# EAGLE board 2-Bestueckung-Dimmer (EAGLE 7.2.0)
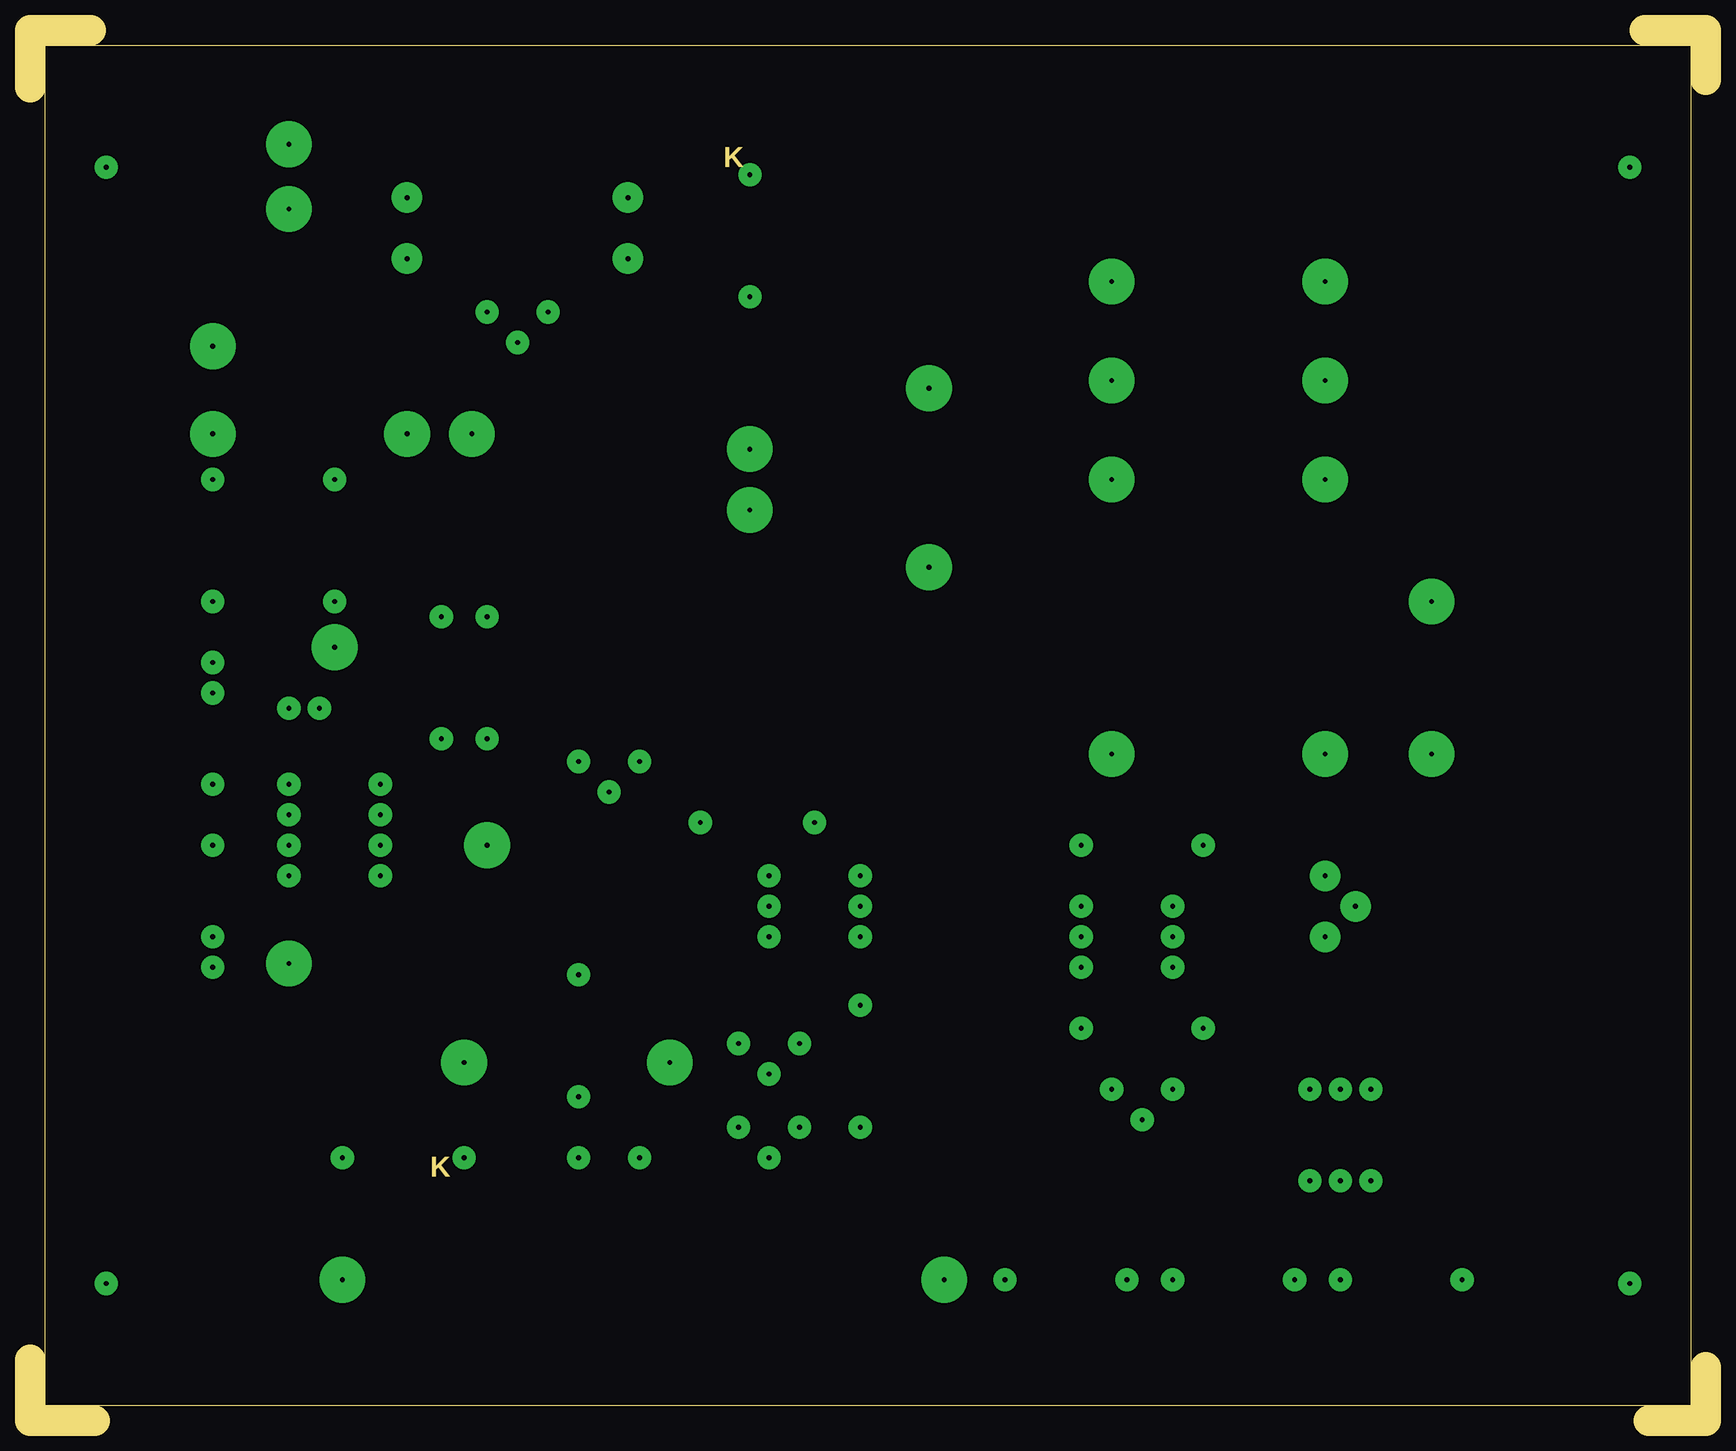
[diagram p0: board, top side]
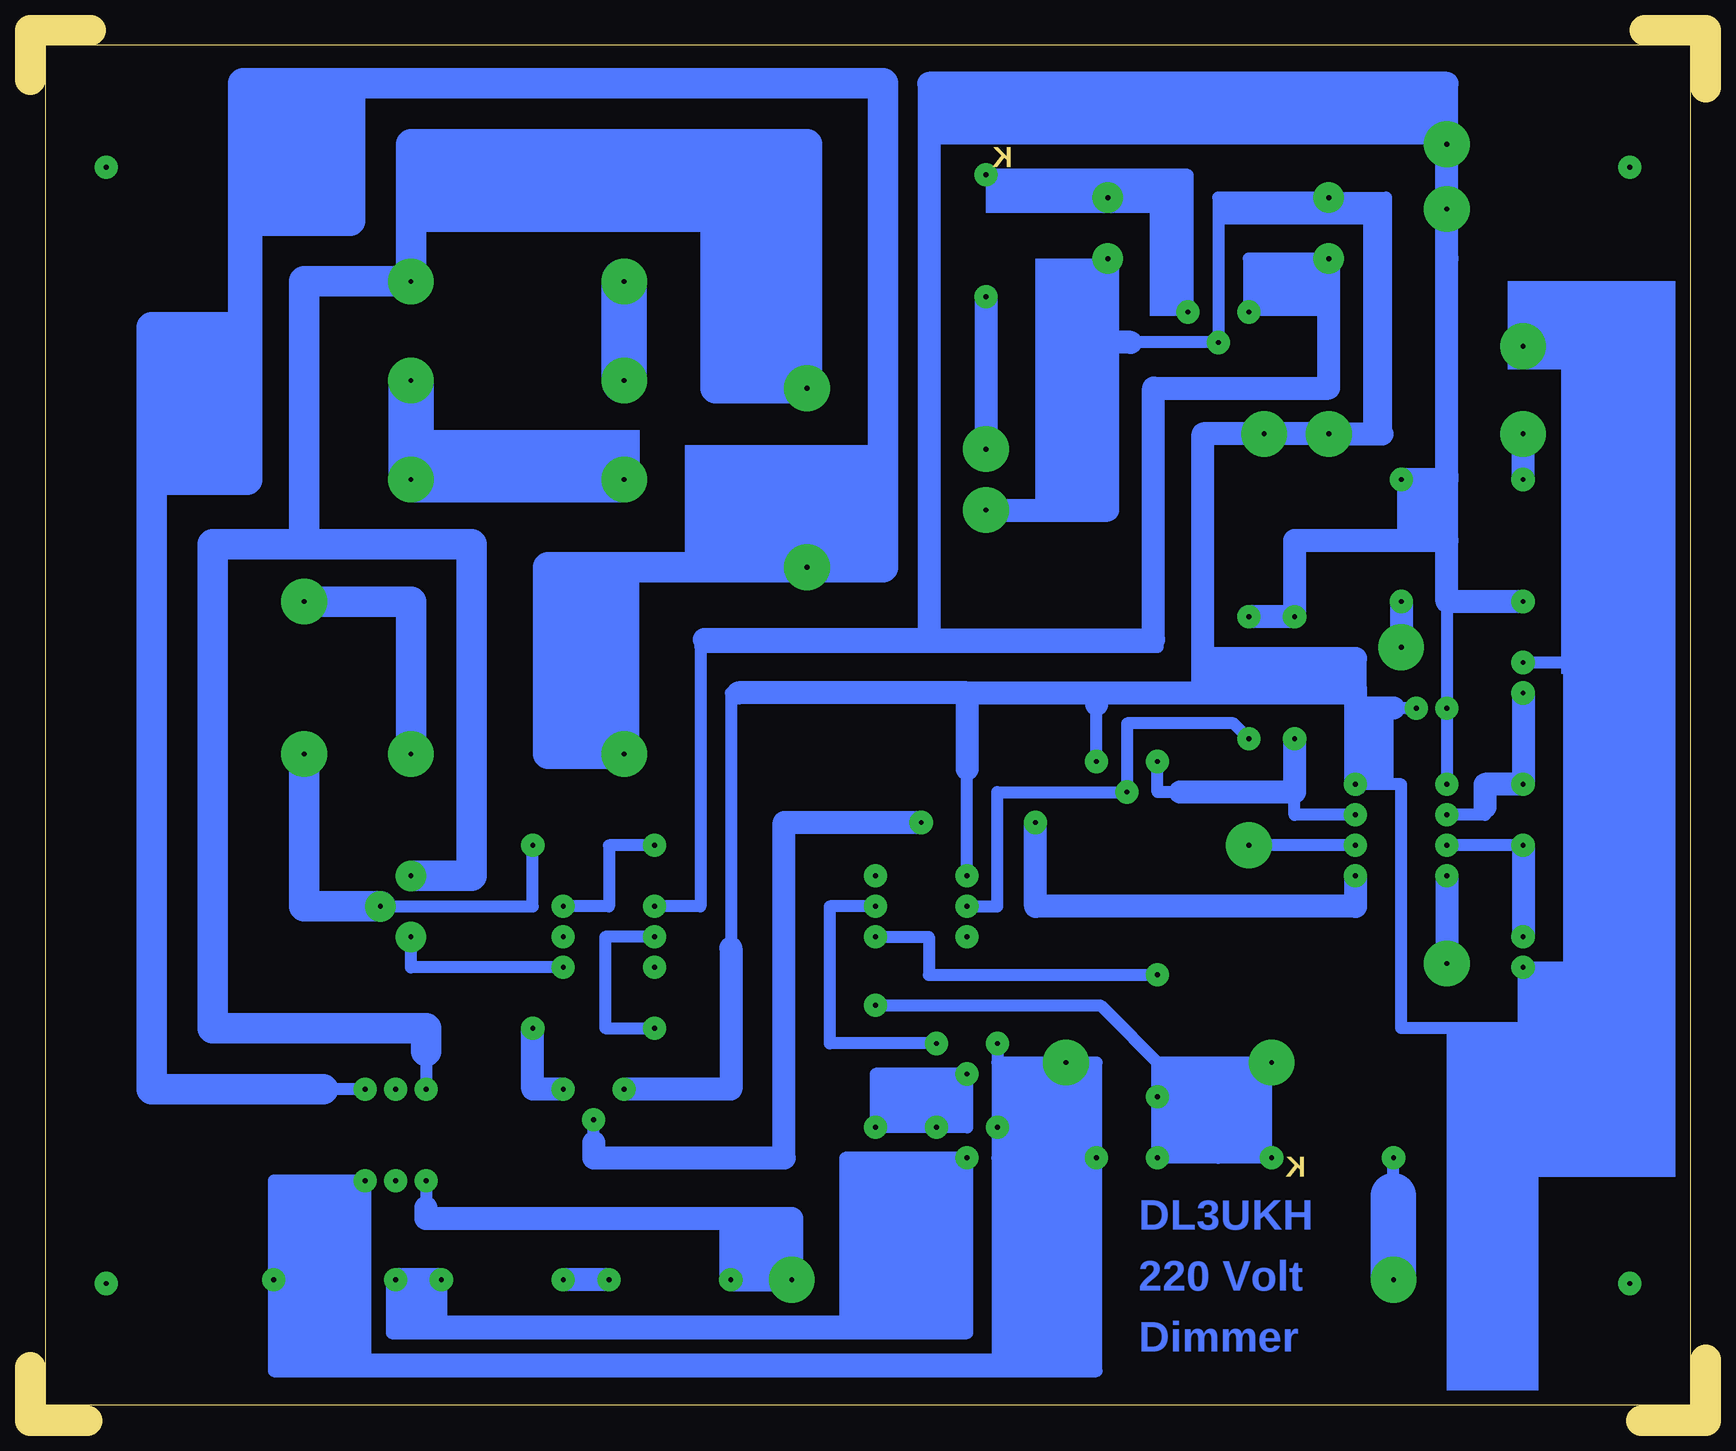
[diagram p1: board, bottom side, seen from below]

Size 139.7 x 115.89 mm. Coordinates in mm from the lower left corner, seen from the top.
Outline: 5.4,0 0.32,0
Outline: 0,0 0,5.08
Outline: 134.94,0 139.7,0 139.7,4.45
Outline: 5.08,115.89 0,115.89 0,111.12
Outline: 139.7,111.76 139.7,115.89
Outline: 134.62,115.89 139.38,115.89
Outline: 1.27,1.27 138.43,1.27 138.43,114.62 1.27,114.62 1.27,1.27
Copper layers (1*16): Top 0.035mm / dielectric 1.5mm / Bottom 0.035mm
Design rules "default": minimum track width 10mil, minimum drill 24mil, track to track 8mil, track to pad 8mil, pad to pad 8mil, via to via 8mil, smd to smd 8mil, copper to edge 40mil, drill to drill 8mil, minimum pad ring 10mil, minimum via ring 8mil, stop-mask expansion 4mil, vias tented up to drill 0mil, thermal gap 10mil

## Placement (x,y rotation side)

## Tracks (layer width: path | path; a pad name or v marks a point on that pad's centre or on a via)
S$1  (via drill 0.4 pad 1.93)
  other vias: 6.35,104.46
S$2  (via drill 0.4 pad 1.93)
  other vias: 133.35,104.46
S$3  (via drill 0.4 pad 1.93)
  other vias: 133.35,11.43
S$4  (via drill 0.4 pad 1.93)
  other vias: 6.35,11.43
S$5  (via drill 0.4 pad 2.54, 0.4 pad 3.81)
  Bottom 1.016: v110.49,42.86 97.79,42.86 97.79,47.94
  Bottom 2.54: v116.84,55.56 116.84,42.86 v110.49,42.86
S$6  (via drill 0.4 pad 1.93, 0.4 pad 2.54, 0.4 pad 3.81)
  Bottom 1.016: v38.1,92.39 38.1,96.84 v31.43,96.84 | 31.43,86.04 45.72,86.04 45.72,64.45 65.09,64.45 | 65.09,64.45 83.82,64.45 83.82,42.86 v87.63,42.86 | 65.09,64.45 65.09,65.09 65.09,111.44 64.77,111.44 | 21.59,111.44 v21.59,106.36 v21.59,100.96 21.59,96.84 | 21.59,78.74 21.59,78.42 | v21.59,53.02 v21.59,59.37 21.59,68.26 21.27,68.26
  Bottom 1.93: v15.24,68.26 21.27,68.26 | 21.59,68.26 21.59,73.34 | 21.59,73.34 34.29,73.34 34.29,66.99 v38.1,66.99 | 21.59,73.34 21.59,78.42 v25.4,78.42 | 21.59,78.74 21.59,96.84 21.59,111.44 64.77,111.44 64.77,65.09 | 64.77,65.09 65.09,65.09 83.5,65.09 | 64.77,65.09 46.04,65.09 46.04,86.04 31.43,86.04 v31.43,96.84
S$7  (via drill 0.4 pad 3.81)
  Bottom 1.016: 107.95,55.25 v107.95,55.56 | 109.54,68.26 v116.84,68.26
  Bottom 2.54: v107.95,55.56 107.95,68.26 108.9,68.26 109.54,68.26
S$8  (via drill 0.4 pad 3.81)
  Bottom 3.81: v90.17,86.68 v90.17,94.93
S$9  (via drill 0.4 pad 1.93, 0.4 pad 2.54, 0.4 pad 3.81)
  Bottom 1.016: 26.04,18.73 v26.04,21.91 | v15.24,78.42 v15.24,82.23 | 47.94,89.85 v40.64,89.85 40.64,101.92 v31.43,101.92 26.67,101.92 26.67,82.23 26.99,82.23 | v31.43,82.23 v36.83,82.23 41.91,82.23 | 80.64,60.64 81.28,60.64 81.28,39.37 | 29.21,59.37 v29.21,53.02 25.4,53.02 25.4,32.7 15.24,32.7 v15.24,37.78 11.43,37.78 11.43,63.18 v15.24,63.18 | 29.21,59.37 29.21,60.64 | v50.8,54.93 50.8,59.69 | v24.13,59.37 26.04,59.37 | 28.89,59.37 29.21,59.37 | v61.6,45.4 61.6,54.29 61.6,60.33 61.91,60.33
  Bottom 1.93: v21.59,45.4 v21.59,38.1 | v15.24,78.42 15.24,82.55 | 61.6,60.64 61.6,54.29 | 61.6,60.64 50.8,60.64 | 50.8,60.64 50.8,59.69 | 50.8,60.64 41.91,60.64 | 41.91,60.64 41.91,60.96 | 41.91,60.96 41.91,63.5 | 41.91,63.5 41.91,82.23 v31.43,82.23 26.99,82.23 | 41.91,60.96 29.21,60.96 | 29.21,60.96 29.21,60.64 | 29.21,60.64 v29.21,53.02 | 26.04,59.37 28.89,59.37 | 29.21,60.96 29.21,63.5 41.91,63.5 | 41.91,60.64 29.21,60.64 | 61.6,60.64 80.64,60.64 | 81.28,39.37 81.28,27.62 v90.17,27.62 | v60.01,75.88 49.85,75.88 49.85,89.85 | 49.85,89.85 v49.85,96.84 | 47.94,89.85 49.85,89.85
  Bottom 3.81: v26.04,11.75 26.04,18.73
S$10  (via drill 0.4 pad 1.93, 0.4 pad 3.81)
  Bottom 1.016: v111.76,27.62 115.25,27.62
  Bottom 1.93: 129.54,78.42 121.92,78.42 121.92,91.12
  Bottom 2.54: 115.25,27.62 129.54,27.62 129.54,33.66 129.54,77.47 129.54,78.42 | 129.54,78.42 121.6,78.42 121.6,100.01 | 121.6,100.01 113.03,100.01 113.03,111.44 | 113.03,111.44 68.58,111.44 68.58,71.12 v74.93,71.12 90.17,71.12 | 90.17,71.12 v90.17,55.56 | v90.17,55.56 90.17,55.25 | v90.17,55.56 96.52,55.56 96.52,71.12 90.17,71.12 | 121.6,100.01 121.92,100.01 | 121.92,100.01 121.92,111.44 113.03,111.44 | 121.92,100.01 121.92,91.12 129.22,91.12 | 129.22,91.12 129.22,78.1 | 129.54,78.42 129.54,91.12 129.22,91.12
S$11  (via drill 0.4 pad 1.93)
  Bottom 1.016: v64.14,31.43 73.02,31.43 73.02,42.86 v69.21,42.86
S$12  (via drill 0.4 pad 3.81)
  Bottom 1.016: 107.95,86.36 v107.95,78.42
  Bottom 3.81: v90.17,78.42 v107.95,78.42 v107.95,86.68 107.95,86.36
S$13  (via drill 0.4 pad 1.93)
  other vias: 97.79,47.94
S$14  (via drill 0.4 pad 1.93)
  Bottom 1.016: v87.63,47.94 91.44,47.94 91.44,42.86 v95.25,42.86
S$15  (via drill 0.4 pad 1.93)
  other vias: 95.25,40.32
S$16  (via drill 0.4 pad 1.93, 0.4 pad 2.54)
  Bottom 1.016: v95.25,37.78 107.95,37.78 v107.95,40.32
S$17  (via drill 0.4 pad 1.93)
  other vias: 87.63,37.78
S$18  (via drill 0.4 pad 1.93)
  Bottom 1.016: v87.63,40.32 91.76,40.32 91.76,32.7 v87.63,32.7
S$19  (via drill 0.4 pad 1.93, 0.4 pad 2.54, 0.4 pad 3.81)
  Bottom 1.016: 122.24,73.02 122.55,73.02 | 106.68,30.8 v106.68,27.62
  Bottom 2.54: v107.95,45.4 102.87,45.4 102.87,73.02 116.84,73.02 | 116.84,73.02 122.24,73.02 | 122.55,73.02 124.46,73.02 124.46,32.7 106.68,32.7 106.68,30.8 | 116.84,73.02 116.84,94.93 v107.95,94.93 107.95,106.36 74.93,106.36 v74.93,86.04 82.55,86.04 82.55,99.69
S$20  (via drill 0.4 pad 3.81)
  other vias: 15.24,89.53
S$21  (via drill 0.4 pad 1.93)
  other vias: 69.21,45.4
S$22  (via drill 0.4 pad 1.93, 0.4 pad 3.81)
  Bottom 1.016: v60.01,80.96 v60.01,93.66
  Bottom 1.93: v60.01,93.66 60.01,80.64
S$23  (via drill 0.4 pad 1.93)
  Bottom 1.93: v29.21,45.4 29.21,42.86 55.88,42.86 v55.88,49.85
S$24  (via drill 0.4 pad 1.93, 0.4 pad 2.54)
  Bottom 1.016: 49.85,103.82 v49.85,101.92 43.18,101.92 v43.18,92.39 43.18,103.82 49.85,103.82 | 49.85,103.82 51.12,103.82 v60.01,103.82
S$25  (via drill 0.4 pad 1.93)
  other vias: 61.6,40.32
S$26  (via drill 0.4 pad 1.93)
  Bottom 1.93: v95.25,27.62 97.79,27.62 v97.79,32.7
S$27  (via drill 0.4 pad 1.93)
  Bottom 1.016: 92.71,23.18 v92.71,25.08
  Bottom 1.93: 92.71,23.18 92.71,21.91 76.83,21.91 76.83,49.85 v65.41,49.85
S$29
  Bottom 2.54: 108.27,68.26 117.16,68.26
S$30  (via drill 0.4 pad 1.93)
  other vias: 109.22,27.62
S$31  (via drill 0.4 pad 1.93)
  Bottom 1.016: v69.21,40.32 64.77,40.32 64.77,37.15 v45.72,37.15
S$32  (via drill 0.4 pad 1.93)
  Bottom 1.016: v38.1,56.83 39.37,58.1 48.26,58.1 v48.26,52.39 59.05,52.39 59.05,42.86 v61.6,42.86
S$33  (via drill 0.4 pad 1.93)
  other vias: 109.22,20
S$34  (via drill 0.4 pad 1.93)
  Bottom 1.016: v111.76,20 111.76,4.45
S$35  (via drill 0.4 pad 1.93, 0.4 pad 3.81)
  Bottom 1.016: v59.05,31.43 59.05,29.84 | 59.05,29.84 v59.05,24.45 59.05,21.91 | 111.76,20 119.38,20 v119.38,11.75 119.38,4.13 59.05,4.13 | 59.05,4.13 50.8,4.13 v50.8,21.91 | 59.05,21.91 53.34,21.91 | 53.34,21.91 v50.8,21.91 | v53.34,29.84 53.34,21.91 | v50.8,21.91 50.8,29.84 59.05,29.84 | 59.05,21.91 59.05,5.08 | 59.05,5.08 59.05,4.13 | 59.05,5.08 119.06,5.08
S$36  (via drill 0.4 pad 1.93, 0.4 pad 3.81)
  Bottom 1.016: v25.4,64.45 v25.4,68.26
  Bottom 1.93: v25.4,68.26 25.4,64.14
S$37  (via drill 0.4 pad 1.93, 0.4 pad 3.81)
  Bottom 1.016: v36.2,21.91 40.64,21.91 | 40.64,21.91 v45.72,21.91 v45.72,26.99 45.72,29.84 40.64,29.84 | v36.2,29.84 40.32,29.84 | 40.32,29.84 40.64,29.84 | 40.64,29.84 40.64,21.91 | 40.32,29.53 40.32,29.84
S$38  (via drill 0.4 pad 1.93)
  other vias: 34.29,66.99
S$39  (via drill 0.4 pad 1.93)
  Bottom 1.93: v91.44,11.75 v95.25,11.75
S$40  (via drill 0.4 pad 1.93)
  Bottom 1.016: v69.21,34.61 50.48,34.61 45.09,29.21
S$41  (via drill 0.4 pad 1.93, 0.4 pad 3.81)
  Bottom 1.016: v106.68,20 106.68,17.78 | 81.28,12.06 v81.28,11.75
  Bottom 1.93: v81.28,11.75 v76.2,11.75 76.2,16.83 81.28,16.83 | 81.28,12.06 81.28,16.83 | 81.28,16.83 82.87,16.83 106.68,16.83 106.68,17.78
S$43  (via drill 0.4 pad 1.93)
  Bottom 1.016: v29.21,50.48 34.29,50.48 34.29,52.39 | 43.82,52.39 45.72,52.39 v45.72,54.93
  Bottom 1.93: v34.29,56.83 34.29,52.39 43.82,52.39
S$45  (via drill 0.4 pad 1.93, 0.4 pad 3.81)
  Bottom 1.016: v29.21,47.94 v38.1,47.94
S$47  (via drill 0.4 pad 1.93)
  Bottom 1.016: v105.41,11.75 105.41,8.26 | 105.41,8.26 105.41,7.3 | 105.41,7.3 71.75,7.3 | 71.75,7.3 61.6,7.3 v61.6,21.91 71.75,21.91 71.75,8.26 | 71.75,8.26 71.75,7.3 | 71.75,8.26 105.41,8.26 | 109.54,11.75 109.54,7.3 105.41,7.3
  Bottom 1.93: v105.41,11.75 v109.22,11.75
S$48  (via drill 0.4 pad 1.93)
  Bottom 1.016: 18.41,51.12 18.41,50.48 v21.59,50.48
  Bottom 1.93: v15.24,60.64 v15.24,53.02 18.41,53.02 18.41,51.12
S$49  (via drill 0.4 pad 1.93)
  Bottom 1.016: v15.24,47.94 v21.59,47.94
  Bottom 1.93: v15.24,47.94 15.24,40.32
S$50  (via drill 0.4 pad 1.93)
  Bottom 1.016: v64.14,24.45 61.6,24.45 v61.6,28.89 69.21,28.89 v69.21,24.45 64.45,24.45
S$55  (via drill 0.4 pad 1.93)
  other vias: 15.24,40.32
(copper drawn outside any net)
  shapes: Bottom area x39

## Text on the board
Bottom: DL3UKH | 220 Volt | Dimmer
Vias: Auf Bestückungsseite gesehen !
Dimension: Cevausit 1,5mm dick | K | alles mit 0,8mm vorgebohrt | K | Aufbohren wie folgt: | K
tOrigins: 1N4148 | 1N4148 | Katode | Anode | + | TIC225 1,0mm | 220V | 470µ/35V | 1000µ/35V | Sicherungshalter 1,5mm | + | Ausg. | Eing. | TIC225 | Netz | an LED | 4Stck. Befestigungsbohr... 3,2mm | Schalter | µA78L05 | an + LED | 1,5K | 10K | Trafo | MT1 | G | 10K | 10K | 3,15A | MT2 | 0,315A | 15p | Sicherung | Sicherung | 47N | E | µA78L05 | 1 | Steckdose | 27K | Brücke | PIC12F675 | 180 | 16Mhz | siehe Beschreibung | BC547c | MT1 | 1 | AN1 | 4N33 | 1 | G | 15p | TIC225 | MOC3021 | 270 | 270 | 3mm LED rt | GP3 | BC547c | 100K | MP | MP | Ausg. | Eing. | (ohne Fassung dargestellt) | E | E | Masse | 1N4148 | 220N | B380C800 | + | - | E | BC547c | BC547c | BC547c | 110K | 10K | 110K | 2 mal 330K | langer | Anschluß- | draht | an +5V | MP | Messpunkte für 7,3Volt DC | C | E | B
